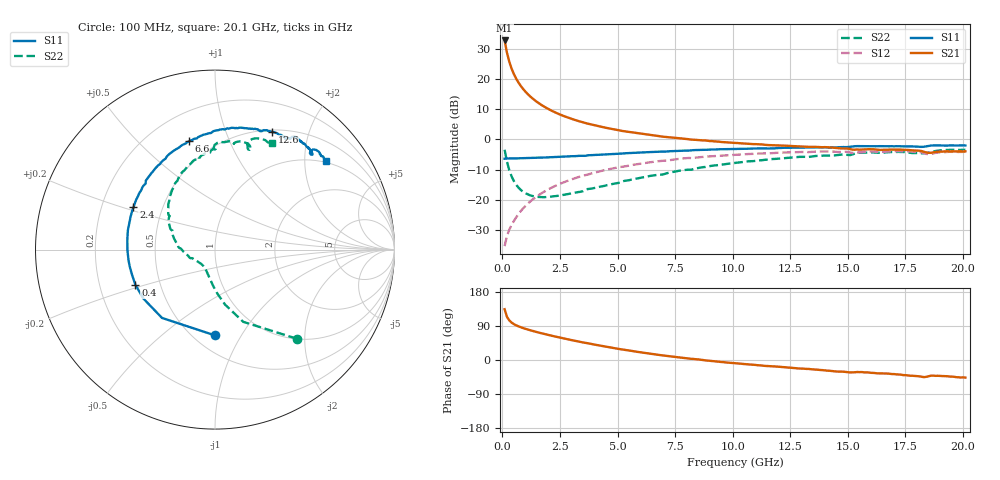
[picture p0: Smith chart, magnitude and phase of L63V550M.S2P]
!  Infineon Technologies AG
! BFR380L3 , PF131585-7, No.6, Th 09.10.01, soldered on pcb-board, measured with PP GSG850
!  Vce=3.5 V,  Ic=50.0 mA
! Common Emitter S-Parameters:  15. November 2001
#  GHz  S  MA  R  50
! f  S11  S21  S12  S22
! GHz  Mag  Ang  Mag  Ang  Mag  Ang  Mag  Ang
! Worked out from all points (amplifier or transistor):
!   201 points, 100 MHz to 20.1 GHz, reference 50 ohm
!   highest |S21| = 32.7 dB at 100 MHz (marker M1)
!   |S21| within 3 dB of that: start of sweep to 175.4 MHz
!   unconditionally stable (mu >= 1): 943.6 MHz to 4.263 GHz
!   at 3.4 GHz: K = 1.02, MAG = 8.3 dB, |S12| = -12.3 dB
!   at 10.1 GHz: K = 0.95, MSG = 2.0 dB, |S12| = -5.1 dB
!   at 20.1 GHz: K = 0.99, MSG = 0.1 dB, |S12| = -4.1 dB
!   S11 on the Smith chart (normalised r, x): 100 MHz: 0.63, -0.78; 400 MHz: 0.36, -0.18; 2.4 GHz: 0.34, +0.22; 6.6 GHz: 0.37, +0.72; 12.6 GHz: 0.52, +1.46; 20.1 GHz: 0.97, +2.55
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0.1  0.4778 -90.1  43.35 134.0  0.01706 61.9  0.6737 -47.5
0.2  0.4818 -127.8  27.41 114.1  0.02502 58.1  0.4321 -68.6
0.3  0.4834 -145.7  19.45 104.7  0.03183 60.6  0.312 -79.6
0.4  0.4848 -156.2  14.93 98.9  0.03795 62.4  0.2456 -86.9
0.5  0.4831 -162.9  12.09 94.7  0.04437 64.6  0.2048 -92.5
0.6  0.4844 -168.5  10.14 91.6  0.05103 66.4  0.1779 -97.2
0.7  0.4855 -172.6  8.743 88.9  0.05788 67.5  0.1592 -101.3
0.8  0.4858 -176.0  7.679 86.5  0.06485 68.3  0.1457 -105.2
1  0.4886 178.3  6.184 82.3  0.0788 69.0  0.1284 -111.8
1.3  0.4929 171.5  4.795 76.9  0.1001 68.9  0.1158 -120.4
1.6  0.4977 165.6  3.925 72.1  0.1212 68.2  0.1111 -127.8
2  0.5051 158.8  3.176 66.1  0.149 66.4  0.1115 -136.2
2.4  0.5124 152.4  2.681 60.5  0.1766 64.2  0.1156 -143.9
3.5  0.5336 136.9  1.907 46.4  0.2503 57.1  0.1386 -160.0
4.9  0.5743 120.5  1.452 30.9  0.3363 47.5  0.1858 179.7
6.6  0.6204 103.6  1.159 15.0  0.4262 35.4  0.2545 159.0
6.8  0.6245 101.6  1.132 13.4  0.4362 33.9  0.2601 156.6
10.1  0.6953 77.5  0.8724 -8.4  0.556 12.1  0.4079 126.0
12.6  0.7291 64.3  0.7746 -20.7  0.6126 -3.4  0.501 105.1
13.5  0.7356 60.3  0.7527 -24.8  0.6225 -8.7  0.5236 98.9
16.8  0.7679 47.8  0.6769 -36.2  0.629 -24.7  0.6148 78.0
20.1  0.7918 38.4  0.6344 -46.3  0.6229 -38.4  0.672 61.8
